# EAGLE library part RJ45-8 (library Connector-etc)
RJ45 Jack Simple RJ45, 8-pin connection - connector for common Cat5, Cat5e, and Cat6 Ethernet cables. Footprint not yet proven in production. Connector sku is PRT-00643; Breakout PCB sku is BOB-00716.
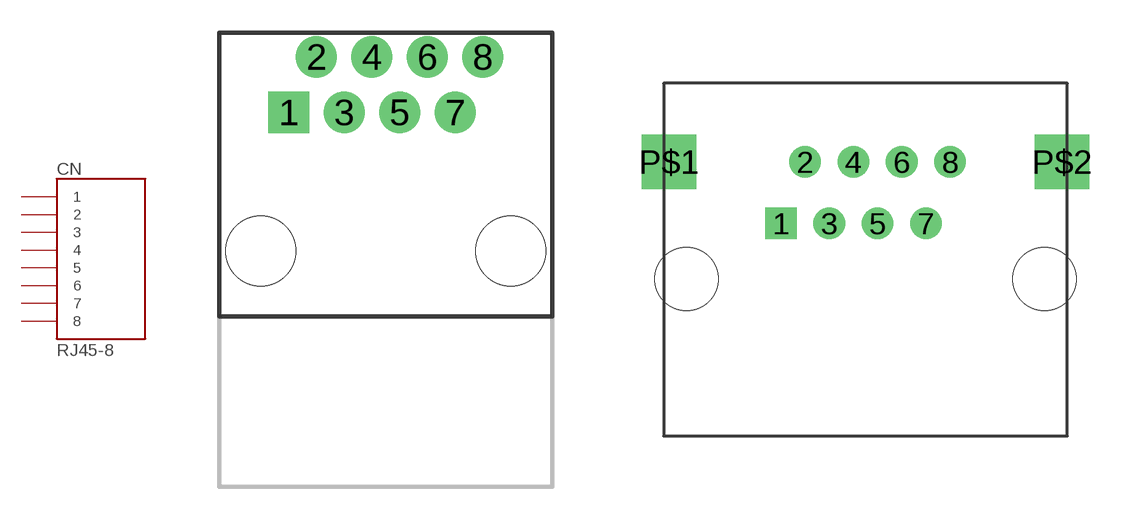
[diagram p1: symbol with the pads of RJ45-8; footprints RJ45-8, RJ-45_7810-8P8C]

Designator prefix CN

## RJ45-8PTH  [RJ45-8]
1  1
2  2
3  3
4  4
5  5
6  6
7  7
8  8

## RJ45-8-7810  [RJ-45_7810-8P8C]
Pads as for RJ45-8

## RJ45-8DIP  [AE-RJ-45-LAN-DIP-A]
Pads as for RJ45-8

## Footprint RJ45-8 (pad centres in mm)
drill 1 pad 1.88 square: 1 -4.445,6.35
drill 1 pad 1.88: 2 -3.175,8.89; 3 -1.905,6.35; 4 -0.635,8.89; 5 0.635,6.35; 6 1.905,8.89; 7 3.175,6.35; 8 4.445,8.89
hole 3.2 at -5.715,0
hole 3.2 at 5.715,0

## Footprint RJ-45_7810-8P8C (pad centres in mm)
CNCでパッド間に1ぽん通すために、少し小さめの穴を設定している。
drill 0.8 square: 1 -3.5,2.3
drill 0.8: 2 -2.5,4.84; 3 -1.5,2.3; 4 -0.5,4.84; 5 0.5,2.3; 6 1.5,4.84; 7 2.5,2.3; 8 3.5,4.84
drill 1.5 square: P$1 -8.125,4.84; P$2 8.125,4.84
hole 2.6 at -7.4,0
hole 2.6 at 7.4,0

## Footprint AE-RJ-45-LAN-DIP-A (pad centres in mm)
RJ-45変換基板 Link: http://akizukidenshi.com/catalog/g/gP-05409/ -- Akitsuki --
drill 1 square: 1 -8.89,8.89
drill 1: 2 -6.35,8.89; 3 -3.81,8.89; 4 -1.27,8.89; 5 1.27,8.89; 6 3.81,8.89; 7 6.35,8.89; 8 8.89,8.89
drill 0.8: P$11 -11.43,-3.81; P$12 11.43,-3.81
